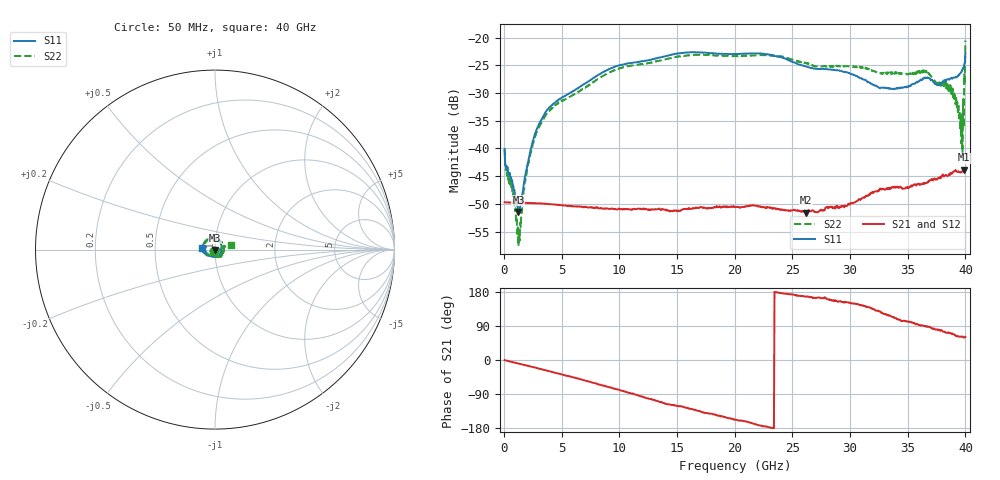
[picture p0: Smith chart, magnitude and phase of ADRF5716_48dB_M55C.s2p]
! Device: ADRF5716
! Description: 30GHz 2-Bit Digital Attenuator
! Frequency: 100 MHz – 30 GHz
! Ports:
! ATTIN  = Port 1
! ATTOUT = Port 2
! State: 48 dB Attenuation selected
! Supply Voltage:
! VDD  =  +3.30 Volts
! VSS  =  -3.30 Volts
! Control Voltages:
! D5 = 3.3V, D6 = 3.3V
! Temperature = -55 C
! Data: Data was collected using a calibrated network analyzer.
!  The reference plane is the package pins of ADRF5716 switch.
! Note: Analog Devices supplies this data as a sample of measured data for this product.
!  Your particular data for this product may vary.
!  Analog Devices reserves the right to change this data at anytime
# HZ S DB R 50
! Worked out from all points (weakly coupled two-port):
!   800 points, 50 MHz to 40 GHz, reference 50 ohm
!   highest |S21| = -43.85 dB at 39.85 GHz (marker M1); lowest = -51.6 dB at 26.2 GHz (marker M2)
!   lowest |S11| = -51.5 dB at 1.25 GHz (marker M3), VSWR 1.01, Z = 49.8 - j0.163 ohm
!   |S11| at or under -10 dB: start of sweep to end of sweep
!   |S22| runs from -57.6 to -20.5 dB; largest |S21 - S12| = 0
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5e7  -40.11 -135.2  -49.72 -0.2  -49.72 -0.2  -40.06 -133.9
7e8  -45.77 176.4  -49.77 -5.2  -49.77 -5.2  -46.93 169.5
1.25e9  -51.47 -142.2  -49.81 -9.3  -49.81 -9.3  -57.65 -141.3
1.45e9  -50.27 -114.5  -49.81 -10.8  -49.81 -10.8  -54.20 -96.2
1.8e9  -45.26 -94.7  -49.82 -13.3  -49.82 -13.3  -45.85 -82.9
2.1e9  -42.15 -89.1  -49.86 -15.5  -49.86 -15.5  -42.58 -81.2
3e9  -35.75 -95.2  -49.93 -22.4  -49.93 -22.4  -36.29 -92.4
4.35e9  -31.85 -111.7  -50.13 -33.0  -50.13 -33.0  -32.33 -111.7
6.75e9  -28.65 -124.7  -50.51 -51.8  -50.51 -51.8  -29.44 -127.4
9.75e9  -25.16 -144.3  -50.99 -77.0  -50.99 -77.0  -25.73 -147.9
1.34e10  -23.63 -166.3  -50.92 -109.5  -50.92 -109.5  -24.20 -173.0
2.005e10  -22.97 149.6  -50.61 -157.4  -50.61 -157.4  -23.33 138.5
2.305e10  -23.11 124.5  -50.64 -178.1  -50.64 -178.1  -23.25 113.1
2.62e10  -25.24 96.2  -51.58 167.5  -51.58 167.5  -24.68 79.6
2.67e10  -25.53 92.5  -51.18 165.5  -51.18 165.5  -25.01 74.0
3.335e10  -29.15 -3.0  -47.27 116.9  -47.27 116.9  -26.49 -8.5
3.655e10  -27.28 -65.6  -46.25 88.4  -46.25 88.4  -25.98 -55.0
3.83e10  -27.78 -104.7  -44.77 72.6  -44.77 72.6  -27.93 -79.7
3.9e10  -27.23 -126.8  -44.13 67.4  -44.13 67.4  -29.77 -84.9
3.965e10  -26.29 -152.4  -44.37 60.7  -44.37 60.7  -39.12 -84.4
3.985e10  -25.47 -166.9  -43.85 60.1  -43.85 60.1  -36.20 3.5
4e10  -22.83 173.8  -43.90 61.1  -43.90 61.1  -20.53 16.2
